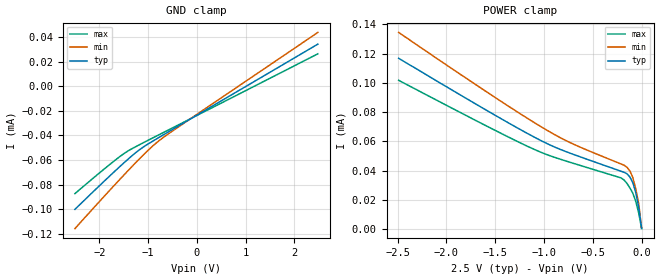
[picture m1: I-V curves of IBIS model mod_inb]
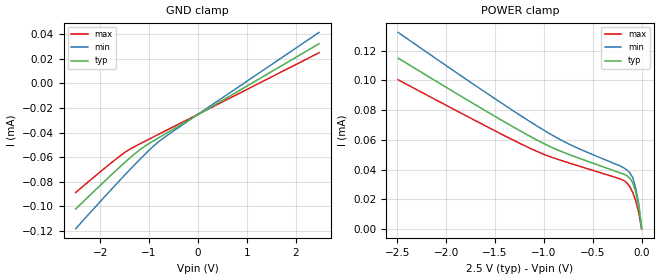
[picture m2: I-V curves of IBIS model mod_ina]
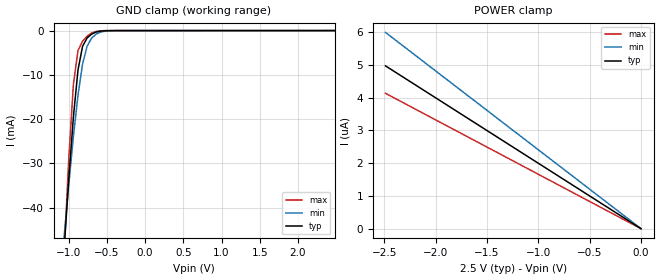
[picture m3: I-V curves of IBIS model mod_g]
| IBIS (I/O, Buffer, Information, Specification) Model, officially
| electronic behavioral standard for Buffer structures of digital pins.
[IBIS ver]  4.2
[File name] rhflvds42_2v5_rev1.ibs
[File Rev]  1.0
[Date]   17 March 2026
[Source]   CAD & Design Services (Catania) - STMicroelectronics
[Notes]
  (Note1) This IBIS model is the model of the product with package
   (Flat16 package elements);
  (Note2) This IBIS model is extracted with nominal 2.5V power supply
   (min:2.30V, typ:2.50V, max:2.70V);
  (Note3) This model has few Notes about the non-monotonicity
   of I-V curves, but they are not indicative of problems
   inside the model;
[Disclaimer]
   Customers are solely responsible for all aspects of their
   own product designs or applications using this IBIS Model.
   STMicroelectronics assumes no liability for Custmer Designs
   and applications associated to this IBIS Model.
   In the use of this IBIS Model Customer shall not modify,
   disassemble, alter this Model in whole or in part.
   If Customers do not accept these terms, the IBIS Model
   may not be used. For any problems or modifications please
   contact STMicroelectronics (www.st.com).
[Copyright] (c) 2026 STMicroelectronics
|   Component RHFLVDS42
[Component] RHFLVDS42
[Manufacturer] STMicroelectronics
[Package]
| variable   typ   min   max
R_pkg   0.0   0.0   0.0
L_pkg   0.0H   0.0H   0.0H
C_pkg   0.0F   0.0F   0.0F
[Pin]  signal_name   model_name   R_pin   L_pin   C_pin
1   1B   mod_inb   0.0   0.0   0.0
2   1A   mod_ina   0.0   0.0   0.0
3   2A   mod_ina   0.0   0.0   0.0
4   2B   mod_inb   0.0   0.0   0.0
5   3B   mod_inb   0.0   0.0   0.0
6   3A   mod_ina   0.0   0.0   0.0
7   4A   mod_ina   0.0   0.0   0.0
8   4B   mod_inb   0.0   0.0   0.0
9   GN   mod_g   0.0   0.0   0.0
10   4Y   mod_y   0.0   0.0   0.0
11   3Y   mod_y   0.0   0.0   0.0
12   GND   GND   0.0   0.0   0.0
13   VCC   POWER   0.0   0.0   0.0
14   2Y   mod_y   0.0   0.0   0.0
15   1Y   mod_y   0.0   0.0   0.0
16   G   mod_g   0.0   0.0   0.0
[Diff pin]  inv_pin   vdiff   tdelay_typ   tdelay_min   tdelay_max
|nA   nB   mV   -   -   -
2   1   100mV   0.0s   0.0s   0.0s
3   4   100mV   0.0s   0.0s   0.0s
6   5   100mV   0.0s   0.0s   0.0s
7   8   100mV   0.0s   0.0s   0.0s
[Package Model]  FE0032_RH_LVDS42
[Define Package Model]  FE0032_RH_LVDS42
[Manufacturer]  STMicroelectronics
[OEM]  STMicroelectronics
[Description]  flat-16
[Number Of Pins]  16
[Pin Numbers]
|Pin Num   Terminal Name
1   | NET1_B1:bw3
2   | NET2_A1:bw4
3   | NET3_A2:bw6
4   | NET4_B2:bw7
5   | NET5_B3:bw9
6   | NET6_A3:bw10
7   | NET7_A4:bw12
8   | NET8_B4:bw13
9   | NET9_GB:bw19
10   | NET10_Y4:bw23
11   | NET11_Y3:bw26
12   | NET12_GND:bw_gnd
13   | NET13_VCC:bw_vcc
14   | NET14_Y2:bw30
15   | NET15_Y1:bw33
16   | NET16_G:bw37
[Model Data]
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[End Model Data]
[End Package Model]
| Models and submodels in the file (4): mod_inb (Input), mod_ina (Input), mod_g (Input), mod_y (3-state)
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|   Model mod_inb
[Model]   mod_inb
Model_type Input
Vinl   =   0.800V
Vinh   =   1.700V
C_comp   11.121pF   10.620pF   11.645pF
[Temperature Range]  25.0000   0.1250k   -55.0000
[Voltage Range]   2.5000V   2.3000V   2.7000V
[GND_clamp]
|Voltage   I(typ)   I(min)   I(max)
-2.5V     -100.2uA   -115.9uA   -87.38uA
-1.84V    -75.04uA   -87uA      -65.44uA
-1.48V    -61.82uA   -71.61uA   -54.43uA
-1.18V    -51.8uA    -59.21uA   -47.68uA
-820mV    -42.71uA   -45.77uA   -40.37uA
-400mV    -32.88uA   -33.75uA   -31.89uA
2.48V     34.23uA    43.77uA    26.34uA
[POWER_clamp]
|Voltage   I(typ)   I(min)   I(max)
-2.49V    116.8uA    134.5uA    101.8uA
-1.5V     77.82uA    89.97uA    67.52uA
-1.02V    60.19uA    69.64uA    52.28uA
-720mV    51.66uA    58.8uA     45.47uA
-210mV    39.61uA    44.58uA    35.06uA
-180mV    38.91uA    43.77uA    33.65uA
-150mV    37.9uA     42.32uA    31.34uA
-120mV    35.7uA     39.85uA    28.24uA
-90mV     31.8uA     35.34uA    24.63uA
-60mV     25.1uA     27.53uA    19.02uA
-30mV     15.2uA     17.52uA    11.21uA
0V        699nA      913nA      401nA
|   Model mod_ina
[Model]   mod_ina
Model_type Input
Vinl   =   0.800V
Vinh   =   1.700V
C_comp   11.121pF   10.620pF   11.645pF
[Temperature Range]  25.0000   0.1250k   -55.0000
[Voltage Range]   2.5000V   2.3000V   2.7000V
[GND_clamp]
|Voltage   I(typ)   I(min)   I(max)
-2.5V     -102.2uA   -118.2uA   -88.78uA
-1.84V    -77.03uA   -89.31uA   -66.84uA
-1.48V    -63.81uA   -73.93uA   -55.83uA
-1.18V    -53.78uA   -61.52uA   -49.09uA
-820mV    -44.69uA   -48.08uA   -41.78uA
-400mV    -34.87uA   -36.06uA   -33.3uA
2.48V     32.24uA    41.45uA    24.94uA
[POWER_clamp]
|Voltage   I(typ)   I(min)   I(max)
-2.49V    114.9uA    132.2uA    100.4uA
-1.5V     75.83uA    87.66uA    66.12uA
-1.02V    58.2uA     67.32uA    50.88uA
-720mV    49.67uA    56.49uA    44.06uA
-240mV    38.32uA    43.08uA    34.27uA
-180mV    36.92uA    41.16uA    32.65uA
-150mV    36.01uA    39.84uA    31.14uA
-120mV    34.3uA     37.85uA    28.54uA
-90mV     31.1uA     34.64uA    24.63uA
-60mV     25.1uA     27.53uA    19.02uA
-30mV     15.2uA     17.52uA    11.21uA
0V        699nA      913nA      401nA
|   Model mod_g
[Model]   mod_g
Model_type Input
Vinl   =   0.800V
Vinh   =   1.700V
C_comp   11.121pF   10.620pF   11.645pF
[Temperature Range]  25.0000   0.1250k   -55.0000
[Voltage Range]   2.5000V   2.3000V   2.7000V
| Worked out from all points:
|   GND clamp passes 1 mA (typ) near -0.71 V on its own axis
[GND_clamp]
|Voltage   I(typ)   I(min)   I(max)
-2.5V     -483.4mA   -366.1mA   -655.1mA
-1.06V    -49.01mA   -46.3mA    -49.88mA
-1V       -33.47mA   -34.75mA   -28.86mA
-940mV    -19.56mA   -24.01mA   -12.18mA
-880mV    -8.954mA   -14.64mA   -4.529mA
-820mV    -3.571mA   -7.568mA   -2.398mA
-760mV    -1.668mA   -3.509mA   -1.253mA
-700mV    -784.6uA   -1.672mA   -536.4uA
-640mV    -327.5uA   -783.7uA   -170.5uA
-580mV    -116.8uA   -326.7uA   -43.27uA
-460mV    -13.5uA    -46.54uA   -6.125uA
2.48V     -39.92nA   434.3nA    -365.3nA
[POWER_clamp]
|Voltage   I(typ)   I(min)   I(max)
-2.49V    4.973uA    5.995uA    4.135uA
-2.19V    4.374uA    5.273uA    3.636uA
-1.47V    2.936uA    3.54uA     2.441uA
0V        24.55pA    1.057nA    21.61pA
